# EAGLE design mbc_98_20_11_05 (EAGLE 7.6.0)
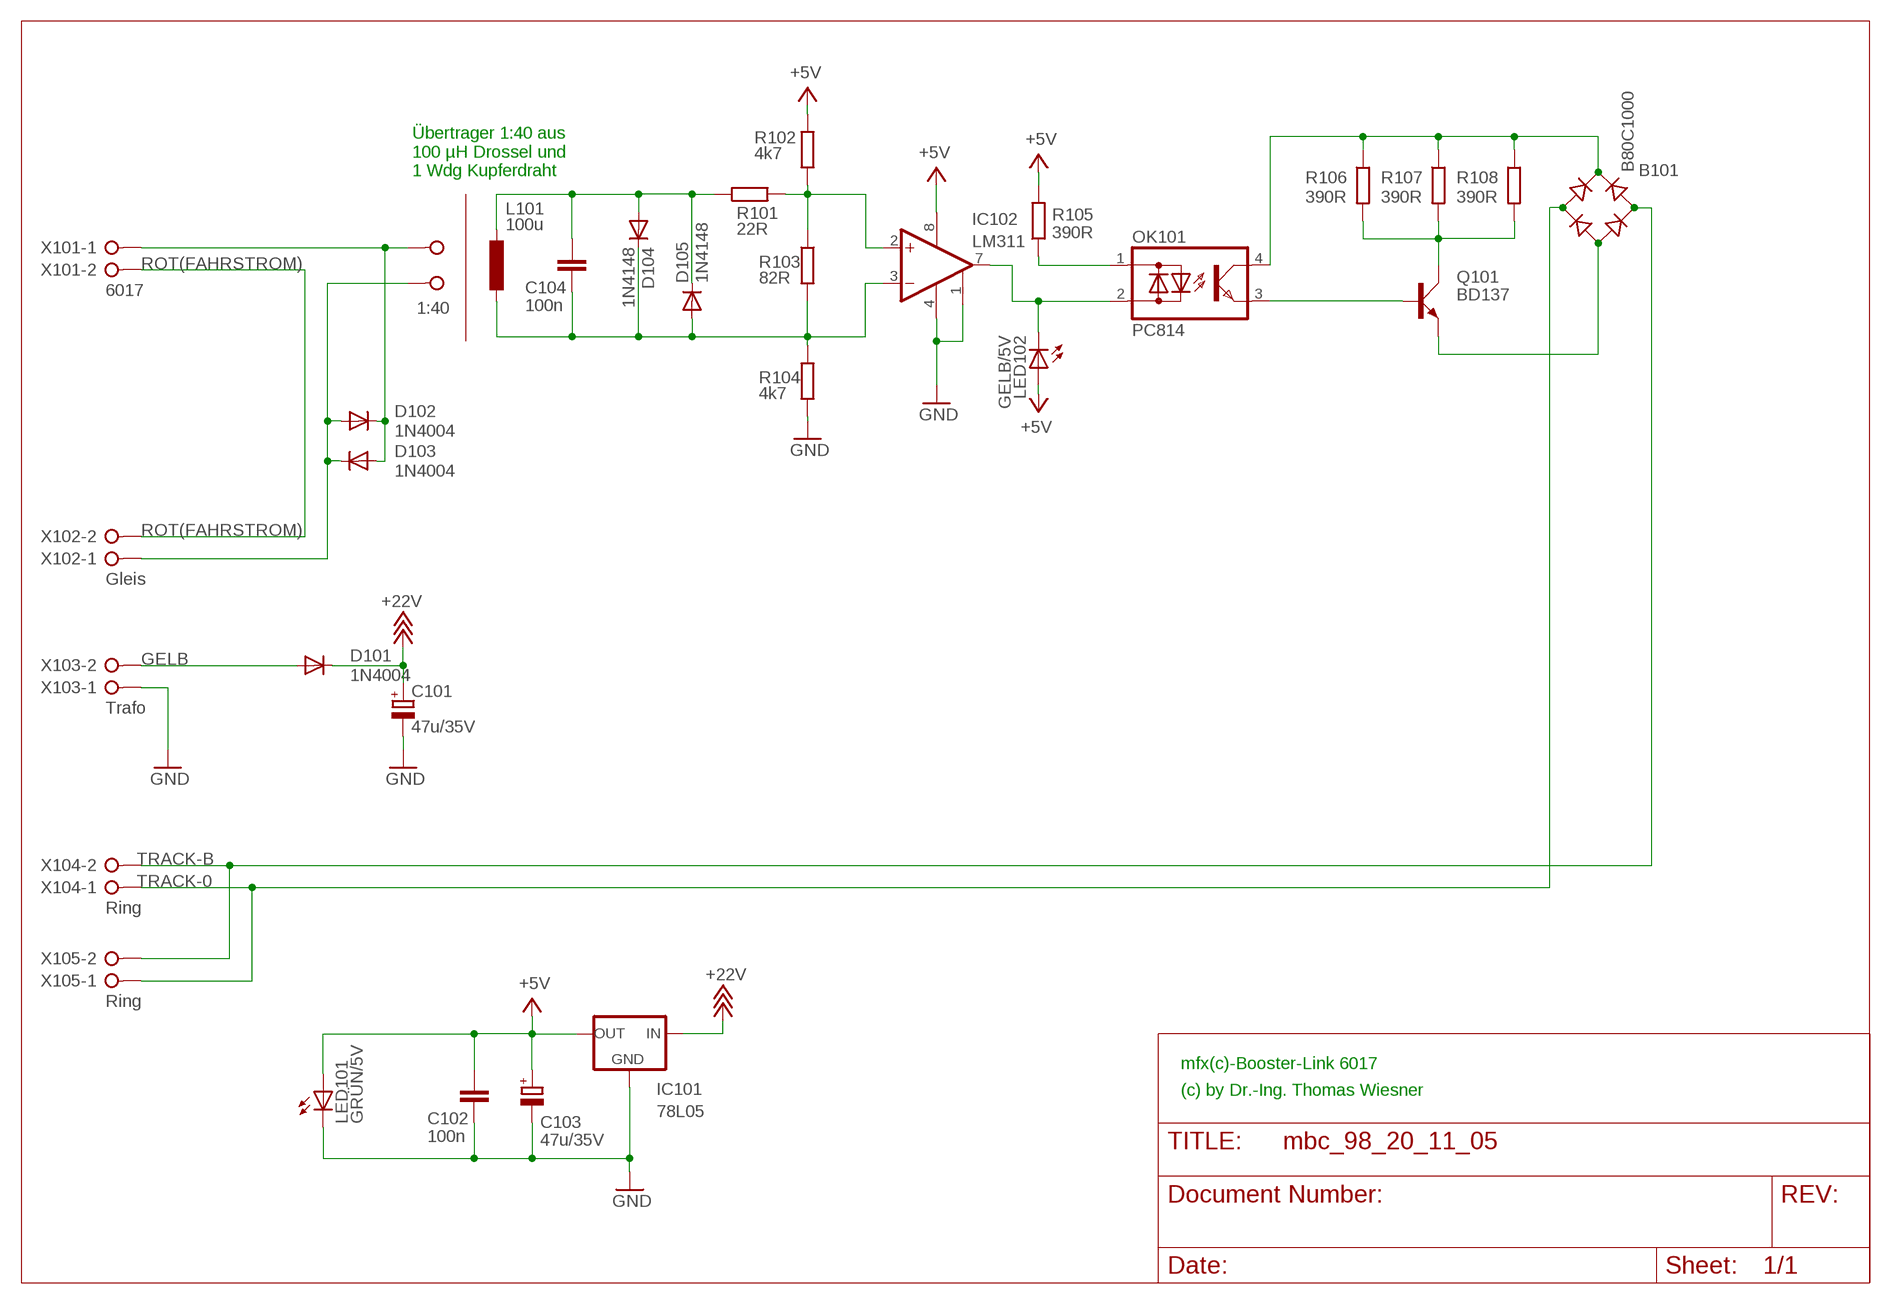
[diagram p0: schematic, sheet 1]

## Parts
B101  B80C1000  RB1A  [RB1A]
C101  47u/35V  CPOL-EUE2.5-7  [E2,5-7]
C102  100n  C-EU025-025X050  [C025-025X050]
C103  47u/35V  CPOL-EUE2.5-7  [E2,5-7]
C104  100n  C-EU025-025X050  [C025-025X050]
D101  1N4004  [DO41-10]
D102  1N4004  [DO41-10]
D103  1N4004  [DO41-10]
D104  1N4148  1N4148DO35-10  [DO35-10]
D105  1N4148  1N4148DO35-10  [DO35-10]
IC101  78L05  78LXX  [78LXX]
IC102  LM311  [DIL08]
L101  100u  L-EU6000-XXX-RC  [6000-XXXX-RC]
LED101  GRÜN/5V  LED3MM  [LED3MM]
LED102  GELB/5V  LED3MM  [LED3MM]
OK101  PC814  [DIL04]
Q101  BD137  BD139  [TO126AV]
R101  22R  R-EU_0207/10  [0207/10]
R102  4k7  R-EU_0207/10  [0207/10]
R103  82R  R-EU_0207/10  [0207/10]
R104  4k7  R-EU_0207/10  [0207/10]
R105  390R  R-EU_0207/10  [0207/10]
R106  390R  R-EU_0207/10  [0207/10]
R107  390R  R-EU_0207/10  [0207/10]
R108  390R  R-EU_0207/10  [0207/10]
TP  1:40  W237-02P  [W237-132]
X101  6017  W237-02P  [W237-132]
X102  Gleis  W237-02P  [W237-132]
X103  Trafo  W237-02P  [W237-132]
X104  Ring  W237-02P  [W237-132]
X105  Ring  W237-02P  [W237-132]

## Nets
+5V: C102.1 C103.+ IC101.OUT IC102.8(V+) LED101.A LED102.A R102.2 R105.2
+18V: C101.+ D101.C IC101.IN ; supply symbol labelled +22V
GELB: D101.A X103.2
GND: C101.- C102.2 C103.- IC101.GND IC102.1(EMIOUT) IC102.4(V-) LED101.K(C) R104.2 X103.1
N$1: OK101.1(AC1) R105.1
N$2: OK101.3(E) Q101.B
N$4: Q101.C R106.2 R107.2 R108.2
N$12: B101.- Q101.E
N$14: C104.2 D104.C D105.A IC102.3(-IN) L101.2 R103.2 R104.1
N$15: IC102.2(+IN) R101.2 R102.1 R103.1
N$16: D102.A D103.C TP.1 X102.1
N$17: B101.+ OK101.4(C) R106.1 R107.1 R108.1
N$19: C104.1 D104.A D105.C L101.1 R101.1
O': D102.C D103.A TP.2 X101.1
PULSE: IC102.7(COLOUT) LED102.K(C) OK101.2(AC2)
ROT(FAHRSTROM): X101.2 X102.2
TRACK-0: B101.AC1 X104.1 X105.1
TRACK-B: B101.AC2 X104.2 X105.2

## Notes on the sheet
- Übertrager 1:40 aus
  100 µH Drossel und 
  1 Wdg Kupferdraht
- mfx(c)-Booster-Link 6017
- (c) by Dr.-Ing. Thomas Wiesner

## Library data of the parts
B101 = rectifier:RB1A: RECTIFIER 1 A
C101 C103 = rcl:CPOL-EU: POLARIZED CAPACITOR, European symbol
C102 C104 = rcl:C-EU: CAPACITOR, European symbol
D101-D103 = diode:1N4004: DIODE
D104 D105 = diode:1N4148: DIODE
IC101 = v-reg:78LXX: VOLTAGE REGULATOR
IC102 = mbc:LM311: DC-Comparator Single
L101 = rcl:L-EU: INDUCTOR, European symbol
LED101 LED102 = led:LED: LED
OK101 = optocoupler:PC814: SHARP OPTO COUPLER; OC_FARNELL: 9707662; OC_NEWARK: unknown
Q101 = transistor-power:BD139: NPN TRANSISTOR
R101-R108 = resistor:R-EU_: RESISTOR, European symbol
TP X101-X105 = con-wago-508:W237-02P: WAGO SREW CLAMP; OC_FARNELL: unknown; OC_NEWARK: unknown

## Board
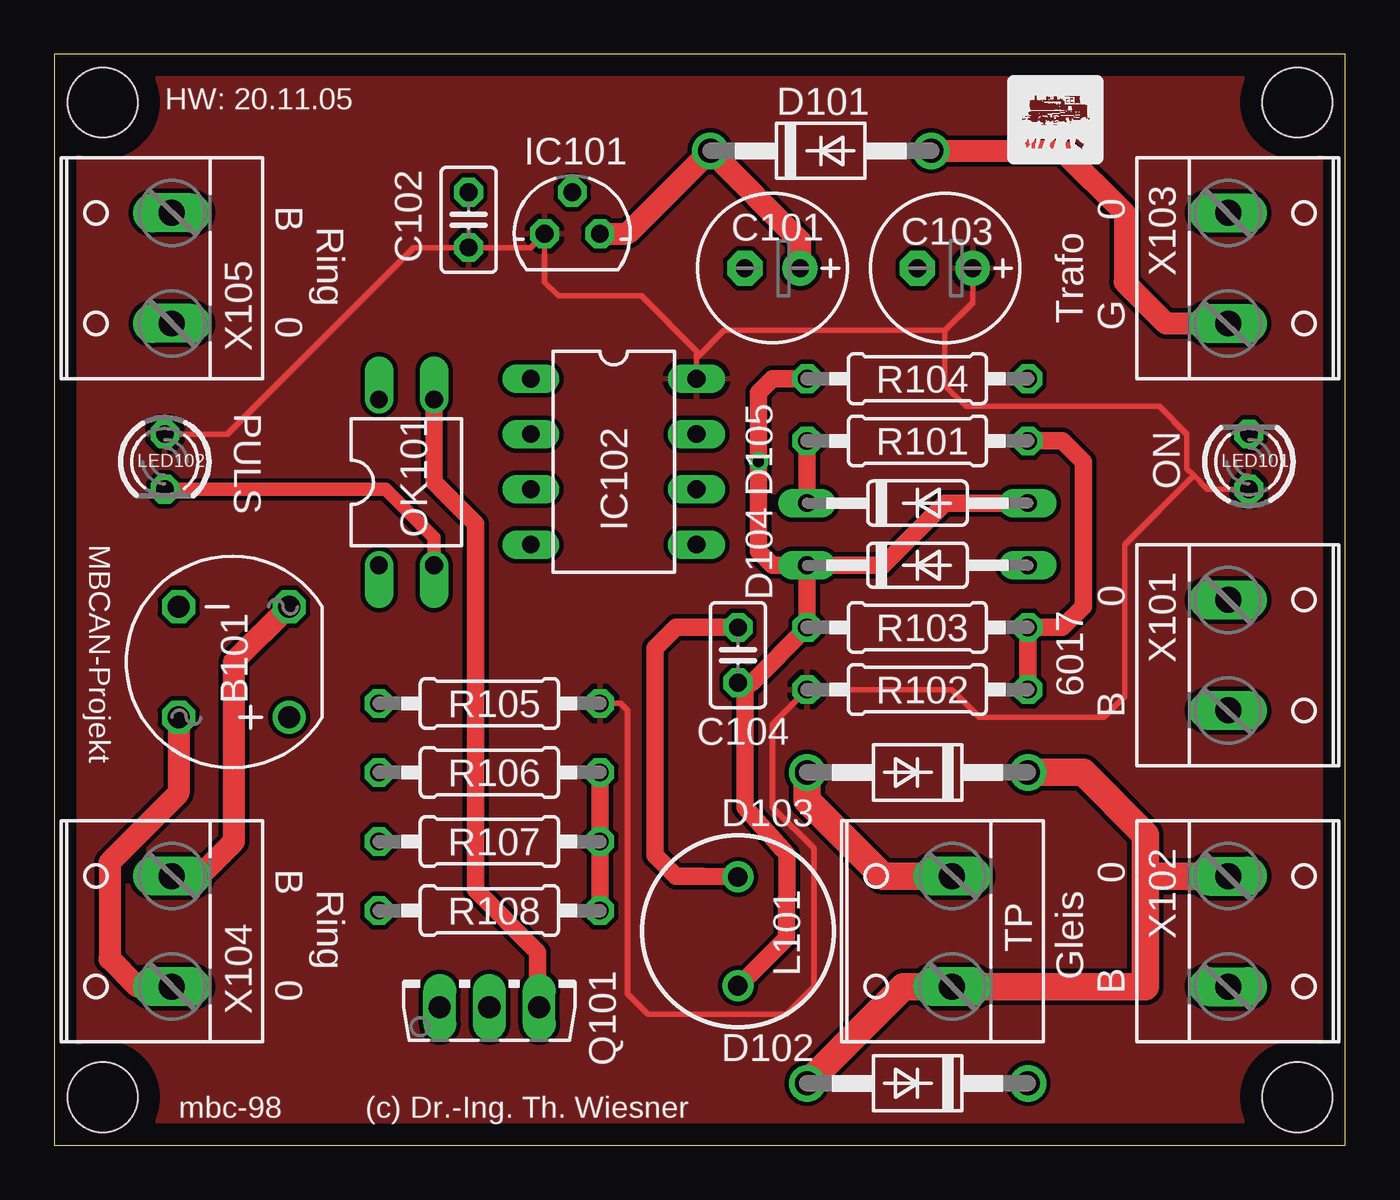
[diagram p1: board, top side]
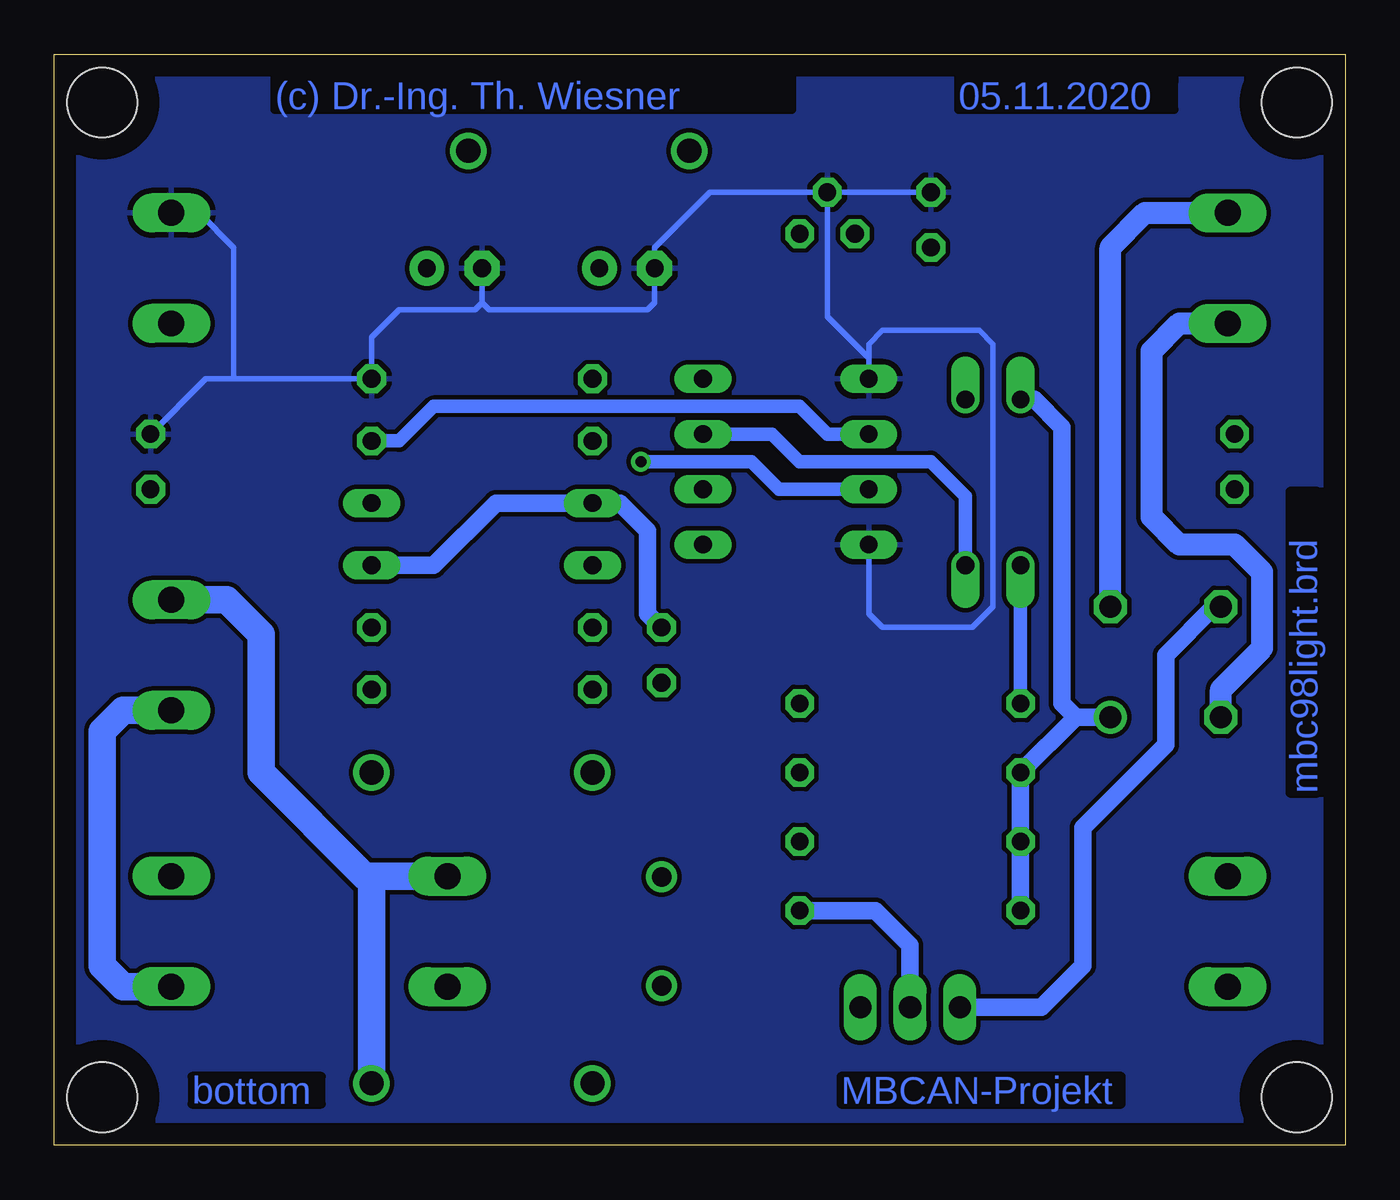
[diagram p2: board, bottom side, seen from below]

Size 59.35 x 50.15 mm. Coordinates in mm from the lower left corner, seen from the top.
Outline: 0,0 59.35,0 59.35,50.15 0,50.15 0,0
Copper layers (1*16): Top 0.035mm / dielectric 1.5mm / Bottom 0.035mm
Design rules "default *": minimum track width 10mil, minimum drill 0.5mm, track to track 8mil, track to pad 8mil, pad to pad 8mil, via to via 8mil, smd to smd 8mil, copper to edge 40mil, drill to drill 8mil, minimum pad ring 10mil, minimum via ring 8mil, stop-mask expansion 4mil, vias tented up to drill 0mil, thermal gap 10mil
Holes 3.2 mm at 2.22,2.22 57.15,2.22 2.22,47.94 57.15,47.94

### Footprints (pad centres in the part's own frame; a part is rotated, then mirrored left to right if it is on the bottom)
RB1A = drill 1.016: + -2.54,2.54 | drill 1.016 octagon: - 2.54,-2.54; AC1 2.54,2.54; AC2 -2.54,-2.54
E2,5-7 = drill 0.813 pad 1.6: + -1.27,0 | drill 0.813 pad 1.6 octagon: - 1.27,0
C025-025X050 = drill 0.813 octagon: 1 -1.27,0; 2 1.27,0
DO41-10 = drill 1.118: A 5.08,0; C -5.08,0
DO35-10 = drill 0.813 long: A 5.08,0; C -5.08,0
78LXX = drill 0.813 octagon: GND 0,1.905; IN 1.27,0; OUT -1.27,0
DIL08 = drill 0.813 long: 1 -3.81,-3.81; 2 -1.27,-3.81; 3 1.27,-3.81; 4 3.81,-3.81; 5 3.81,3.81; 6 1.27,3.81; 7 -1.27,3.81; 8 -3.81,3.81
6000-XXXX-RC = drill 0.9 pad 1.422: 1 -2.5,0; 2 2.5,0
LED3MM = drill 0.813 octagon: A -1.27,0; K 1.27,0
DIL04 = drill 0.813 offset: 1 -1.27,-3.81; 2 1.27,-3.81; 3 1.27,3.81; 4 -1.27,3.81
TO126AV = drill 1.016 long: B 2.286,-1.27; C 0,-1.27; E -2.286,-1.27
0207/10 = drill 0.813 octagon: 1 -5.08,0; 2 5.08,0
W237-132 = drill 1.194 long: 1 -2.54,-0.635; 2 2.54,-0.635

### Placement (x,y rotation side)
B101  8.26,22.23 180 top
C101  33.02,40.32 180 top
C102  19.05,42.55 90 top
C103  40.96,40.32 180 top
C104  31.43,22.54 270 top
D101  35.24,45.72 0 top
D102  39.69,2.86 180 top
D103  39.69,17.14 180 top
D104  39.69,26.67 0 top
D105  39.69,29.53 0 top
IC101  23.81,41.91 0 top
IC102  25.72,31.43 270 top
L101  31.43,9.84 270 top
LED101  54.93,31.43 90 top
LED102  5.08,31.43 270 top
OK101  16.19,30.48 0 top
Q101  20,7.62 0 top
R101  39.69,32.38 0 top
R102  39.69,20.95 180 top
R103  39.69,23.81 180 top
R104  39.69,35.24 0 top
R105  20,20.32 0 top
R106  20,17.14 0 top
R107  20,13.97 0 top
R108  20,10.79 0 top
TP  40.64,9.84 90 top
X101  54.61,22.54 270 top
X102  54.61,9.84 270 top
X103  54.61,40.32 270 top
X104  4.76,9.84 90 top
X105  4.76,40.32 90 top

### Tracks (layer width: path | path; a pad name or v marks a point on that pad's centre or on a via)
+5V
  Top 0.254: LED102.A 7.94,32.7 16.51,41.27 C102.1 21.91,41.27 IC101.OUT 22.54,39.69 23.18,39.05 26.99,39.05 29.53,36.51 29.53,36.2 | 29.53,36.2 IC102.8 | C103.+ 42.23,38.73 40.96,37.47 | 40.96,37.47 30.8,37.47 29.53,36.2 | LED101.A 53.02,30.16 52.39,30.8 | 52.39,30.8 52.07,31.11 52.07,32.7 50.8,33.97 41.91,33.97 40.96,34.92 40.96,37.47 | R105.2 26.04,20.32 26.35,20 26.35,6.99 27.3,6.03 33.66,6.03 34.92,7.3 34.92,13.65 33.02,15.56 33.02,19.37 R102.2 41.27,20.95 42.55,19.68 48.26,19.68 49.21,20.64 49.21,27.62 52.39,30.8
  pour Top: 0,50.16 59.37,50.16 59.37,0 0,0
+18V
  Top 1.016: C101.+ 34.29,41.59 D101.C 26.35,41.91 IC101.IN
GELB
  Top 1.016: D101.A 46.35,45.72 49.21,42.86 49.21,39.69 51.12,37.78 X103.2
GND
  Bottom 0.254: C102.2 IC101.GND | IC101.GND 29.21,43.81 31.75,41.27 C101.- 31.75,38.73 32.07,38.42 39.37,38.42 39.69,38.73 | 39.69,38.73 C103.- | 39.69,38.73 40.01,38.42 43.5,38.42 44.77,37.15 R104.2 51.12,35.24 | 51.12,35.24 52.39,35.24 LED101.K | X103.1 52.7,42.86 51.12,41.27 51.12,35.24 | IC101.GND 23.81,38.1 21.91,36.2 IC102.1 21.91,36.83 21.27,37.47 16.83,37.47 16.19,36.83 16.19,24.77 17.14,23.81 21.27,23.81 21.91,24.45 IC102.4
  pour Bottom: 0,50.16 59.37,50.16 59.37,0 0,0
N$1
  Bottom 0.61: R105.1 OK101.1
N$2
  Top 0.813: OK101.3 17.46,30.48 19.37,28.57 19.37,11.75 22.23,8.89 22.23,6.41 Q101.B
N$4
  Top 0.813: R106.2 R107.2 R108.2
  Bottom 0.813: Q101.C 20,9.21 21.59,10.79 R108.2
N$12
  Bottom 0.813: B101.- 6.03,24.77 8.26,22.54 8.26,18.41 12.06,14.61 12.06,8.26 13.97,6.35 Q101.E
N$14  (via drill 0.5)
  Top 0.813: D105.A 40.96,29.53 38.1,26.67 D104.C | D104.C R103.2 32.07,21.27 C104.2 31.75,20.95 31.75,15.56 33.7,13.38 33.66,9.53 31.47,7.34 L101.2 | D104.C 33.02,26.67 32.38,27.3 v32.38,31.43 32.38,34.61 33.02,35.24 R104.1
  Bottom 0.61: IC102.3 26.04,30.16 27.3,31.43 v32.38,31.43
N$15
  Top 0.813: R101.2 46.35,32.38 47.31,31.43 47.31,24.77 46.35,23.81 R103.1 R102.1
  Bottom 0.61: IC102.2 23.81,32.7 25.08,33.97 41.91,33.97 43.5,32.38 R101.2
N$16
  Top 1.27: 50.16,12.38 50.16,7.3 TP.1 39.05,7.3 D102.A | 50.16,12.38 50.16,14.29 47.31,17.14 D103.C | X102.1 50.16,12.38
N$17
  Bottom 0.813: B101.+ 12.38,19.68 | 12.38,19.68 R106.1 R107.1 R108.1 | OK101.4 14.29,34.29 13.02,33.02 13.02,20.32 12.38,19.68
N$19
  Top 0.813: C104.1 28.57,23.81 27.62,22.86 27.62,13.34 28.57,12.38 29.8,12.38 L101.1 | R101.1 D105.C
  Bottom 0.813: D104.A 41.91,26.67 39.05,29.53 D105.C 33.34,29.53 32.07,28.26 32.07,24.45 C104.1
O'
  Top 1.27: D103.A 34.61,15.88 38.1,12.38 TP.2
  Bottom 1.27: 44.77,12.38 45.09,12.38 49.85,17.14 49.85,23.5 51.44,25.08 X101.1 | 44.77,12.38 TP.2 | D102.C 44.77,12.38
PULSE
  Top 0.61: LED102.K 15.24,30.16 17.46,27.94 OK101.2
  Bottom 0.61: IC102.7 26.35,32.7 25.08,31.43 19.05,31.43 17.46,29.84 OK101.2
ROT(FAHRSTROM)
  Bottom 1.27: X101.2 56.2,20 57.15,19.05 57.15,8.26 56.2,7.3 X102.2
TRACK-0
  Top 1.016: B101.AC1 5.71,16.19 2.54,13.02 2.54,8.57 3.81,7.3 X104.1
  Bottom 1.016: B101.AC1 5.71,20.95 3.81,22.86 3.81,26.35 5.08,27.62 7.62,27.62 8.89,28.89 8.89,36.51 7.62,37.78 X105.1
TRACK-B
  Top 1.016: B101.AC2 8.26,22.23 8.26,13.97 6.67,12.38 X104.2
  Bottom 1.016: B101.AC2 10.79,41.27 9.21,42.86 X105.2

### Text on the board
Bottom: 05.11.2020 | (c) Dr.-Ing. Th. Wiesner | mbc98light.brd | MBCAN-Projekt | bottom
tNames: HW: 20.11.05 | B | 0 | Ring | 0 | Trafo | G | PULS | ON | MBCAN-Projekt | 0 | 6017 | B | B | Ring | 0 | 0 | Gleis | B | mbc-98 | (c) Dr.-Ing. Th. Wiesner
